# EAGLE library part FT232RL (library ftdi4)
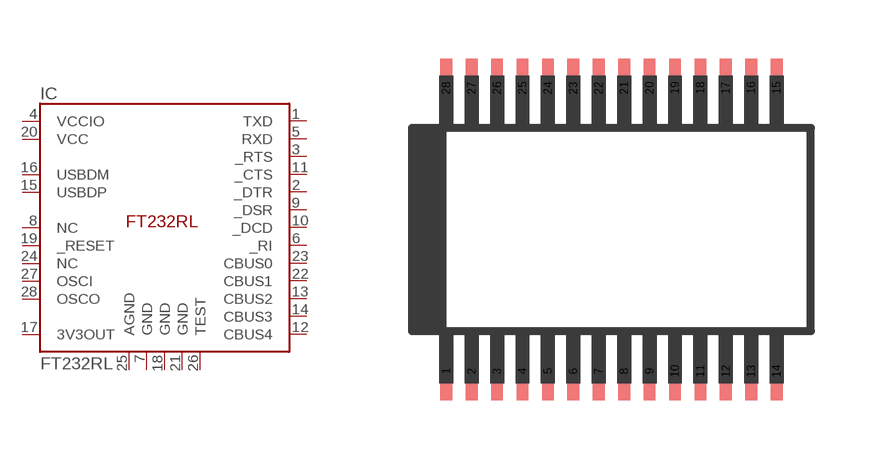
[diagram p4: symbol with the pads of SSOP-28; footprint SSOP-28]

Designator prefix IC

## FT232RL  [SSOP-28]
1  TXD  out
2  _DTR  in
3  _RTS  out
4  VCCIO  pwr
5  RXD  in
6  _RI  in
7  GND  pwr
8  NC  nc
9  _DSR  in
10  _DCD  in
11  _CTS  in
12  CBUS4
13  CBUS2
14  CBUS3
15  USBDP
16  USBDM
17  3V3OUT  out
18  GND  pwr
19  _RESET  in
20  VCC  pwr
21  GND  pwr
22  CBUS1
23  CBUS0
24  NC  nc
25  AGND  pwr
26  TEST
27  OSCI  in
28  OSCO  out

## Footprint SSOP-28 (pad centres in mm)
Shrink Small Outline Package: SSOP-28
smd 0.3 x 1.5: 1 -4.225,-3.625; 2 -3.575,-3.625; 3 -2.925,-3.625; 4 -2.275,-3.625; 5 -1.625,-3.625; 6 -0.975,-3.625; 7 -0.325,-3.625; 8 0.325,-3.625; 9 0.975,-3.625; 10 1.625,-3.625; 11 2.275,-3.625; 12 2.925,-3.625; 13 3.575,-3.625; 14 4.225,-3.625; 15 4.225,3.625; 16 3.575,3.625; 17 2.925,3.625; 18 2.275,3.625; 19 1.625,3.625; 20 0.975,3.625; 21 0.325,3.625; 22 -0.325,3.625; 23 -0.975,3.625; 24 -1.625,3.625; 25 -2.275,3.625; 26 -2.925,3.625; 27 -3.575,3.625; 28 -4.225,3.625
